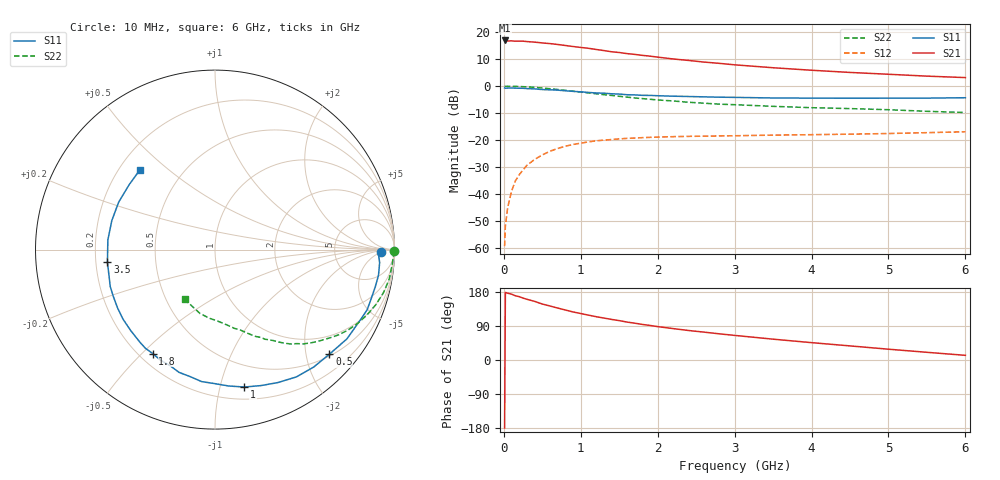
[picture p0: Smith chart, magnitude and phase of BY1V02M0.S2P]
! SIEMENS Small Signal Semiconductors
! BFY420
! Si NPN RF SIEGET Grounded Emitter Transistor in MICRO-X
! VCE = 1 V  IC = 2 mA
! Common Emitter S-Parameters:  October  1996
# GHz  S  MA  R  50
!  f  S11  S21  S12  S22
! GHz  MAG  ANG  MAG  ANG  MAG  ANG  MAG  ANG
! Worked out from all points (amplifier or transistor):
!   36 points, 10 MHz to 6 GHz, reference 50 ohm
!   highest |S21| = 16.9 dB at 10 MHz (marker M1)
!   |S21| within 3 dB of that: start of sweep to 1.124 GHz
!   unconditionally stable (mu >= 1): 3.977 GHz to end of sweep
!   at 250 MHz: K = 0.06, MSG = 23.8 dB, |S12| = -31.0 dB
!   at 1.4 GHz: K = 0.32, MSG = 16.2 dB, |S12| = -19.7 dB
!   at 6 GHz: K = 1.27, MAG = 6.9 dB, |S12| = -16.9 dB
!   S11 on the Smith chart (normalised r, x): 10 MHz: 24, -5; 500 MHz: 0.54, -2.48; 1 GHz: 0.30, -1.19; 1.8 GHz: 0.25, -0.54; 3.5 GHz: 0.25, -0.05; 6 GHz: 0.28, +0.40
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0.01  0.9236 -1.0  6.977 -179.5  0.0011 90.5  0.996 -0.5
0.02  0.9122 -2.0  6.914 178.4  0.0026 88.2  0.9933 -0.9
0.05  0.9201 -4.5  6.823 176.2  0.0057 87.8  0.9947 -2.4
0.1  0.9221 -8.9  6.858 173.8  0.0114 86.2  0.9904 -4.9
0.15  0.9168 -13.0  6.766 169.5  0.0177 81.3  0.9863 -7.3
0.2  0.9125 -17.1  6.778 167.1  0.023 80.8  0.9847 -9.6
0.25  0.9116 -21.6  6.771 163.4  0.0283 76.6  0.9753 -12.1
0.4  0.8875 -34.1  6.499 154.7  0.0441 69.8  0.9472 -18.9
0.5  0.8638 -42.4  6.279 147.7  0.0535 65.4  0.922 -23.3
0.7  0.8419 -57.4  5.879 137.1  0.0703 56.7  0.8661 -31.2
0.9  0.7998 -71.3  5.392 126.8  0.0835 49.0  0.8044 -37.8
1  0.7831 -77.9  5.18 122.6  0.0881 45.9  0.7743 -41.0
1.1  0.7636 -84.3  4.999 118.4  0.0932 43.0  0.7472 -44.0
1.4  0.7209 -101.1  4.314 107.1  0.103 34.9  0.6727 -51.4
1.6  0.6927 -111.4  3.985 100.1  0.1081 30.6  0.6259 -55.4
1.8  0.675 -120.9  3.701 93.9  0.1115 27.2  0.5876 -58.9
2.2  0.6509 -136.3  3.175 82.9  0.1163 21.4  0.5313 -65.3
2.8  0.6238 -155.3  2.635 69.1  0.1199 15.9  0.4635 -73.4
3.5  0.6033 -173.4  2.184 55.0  0.1241 11.6  0.4225 -81.5
4.5  0.5972 164.2  1.789 37.2  0.1293 7.6  0.3838 -94.5
5.5  0.5997 142.8  1.528 20.3  0.1379 5.0  0.342 -111.2
6  0.6098 133.4  1.437 12.3  0.1431 3.7  0.3252 -121.3
